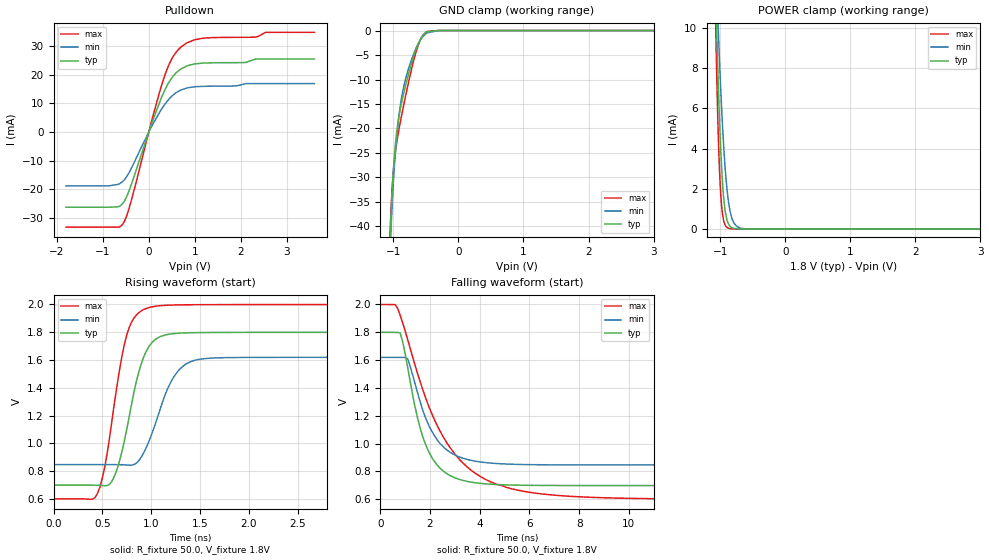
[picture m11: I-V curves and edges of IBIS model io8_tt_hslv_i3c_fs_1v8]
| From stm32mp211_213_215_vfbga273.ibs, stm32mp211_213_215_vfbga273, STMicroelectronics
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[Model]   io8_tt_hslv_i3c_fs_1v8
Model_type I/O_open_drain
Polarity   Non-Inverting
Enable   Active-Low
| CAP_THRESHOLD on pad IOTT is "UDTCAPC" :
| Rising=30.0% of vddiov33m   Falling=70.0% of vddiov33m
| C_comp min and max val. don't necessarily correlate with the min and max pvt
| but are the smallest and greatest pad capacitance found.
| var   typ   min   max
C_comp   1.23130pF  1.11695pF  1.38090pF
|C_comp_pulldown   1.23130pF  1.11695pF  1.38090pF
Vinl = 810.0mV
Vinh = 1.0V
Vmeas = 900.0mV   | Reference voltage for timing measurements
Cref  = 50.0pF   | Timing specification test load capacitance value
Rref  = 1.0MOhm   | Timing specification test load resistance value
Vref  = 990.0mV   | Timing specification test load voltage
[Model Spec]
| TIME_THRESHOLD on pin ZIV08M is "CMOS" :
| Rising=50.0% of vddv08m   Falling=50.0% of vddv08m
Vinl 675.70000mV 623.70000mV 735.70000mV
Vinh 1.12730V 1.01130V 1.24930V
| variable   typ   min   max
[Temperature Range] 25.0 125.0 -40.0
| variable   typ   min   max
[Voltage Range] 1.8V 1.62V 2.0V
| variable   typ   min   max
[POWER Clamp Reference] 1.8V 1.62V 2.0V
| variable   typ   min   max
[GND Clamp Reference] 0V 0V 0V
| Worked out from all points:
|   slope of the pulldown table from 0 to 0.27 V, typ, clamps not added: 22.9 ohm
|   GND clamp passes 1 mA (typ) near -0.55 V on its own axis
|   POWER clamp passes 1 mA (typ) near -0.93 V on its own axis
|   rising waveform, R_fixture 50.0, V_fixture 1.8V: 20-80 % time 209ps typ, 251ps min, 191ps max; typ from 0.698 V to 1.8 V
|   falling waveform, R_fixture 50.0, V_fixture 1.8V: 20-80 % time 948ps typ, 1.06ns min, 2.08ns max; typ from 1.8 V to 0.698 V
[POWER Clamp]
-1.8V     152.1mA    105.6mA    221.1mA
-1.07V    12.07mA    13.61mA    10.38mA
-1.05V    9.569mA    11.75mA    7.248mA
-1.03V    7.339mA    9.993mA    4.743mA
-1.01V    5.42mA     8.357mA    2.898mA
-990mV    3.841mA    6.859mA    1.662mA
-970mV    2.609mA    5.513mA    906.4uA
-940mV    1.358mA    3.806mA    344.1uA
-880mV    308.2uA    1.548mA    45.5uA
-790mV    28.46uA    298.8uA    2.106uA
-610mV    211.8nA    7.522uA    9.52nA
3.6V      0A         0A         0A
[GND Clamp]
-1.8V     -1.222A    -1.193A    -1.238A
-1.05V    -42.33mA   -45.55mA   -41.2mA
-1.04V    -38.89mA   -42.1mA    -37.88mA
-1.03V    -35.83mA   -38.98mA   -35.06mA
-1.01V    -30.7mA    -33.54mA   -30.61mA
-970mV    -23.47mA   -25.17mA   -24.97mA
-920mV    -18.06mA   -18.06mA   -20.63mA
-870mV    -14.51mA   -13.44mA   -17.13mA
-780mV    -9.532mA   -8.354mA   -11.38mA
-650mV    -3.743mA   -3.581mA   -4.327mA
-490mV    -324.1uA   -556uA     -259.6uA
3.6V      66.06nA    2.767uA    18.5nA
| variable   typ   min   max
[Pullup Reference] 1.8V 1.62V 2.0V
| variable   typ   min   max
[Pulldown Reference] 0V 0V 0V
[Pulldown]
-1.8V     -26.25mA   -18.79mA   -33.2mA
-680mV    -26.1mA    -18.31mA   -33.2mA
-550mV    -24.6mA    -16.98mA   -31.75mA
-400mV    -19.26mA   -13.3mA    -25.07mA
70mV      3.286mA    2.202mA    4.389mA
320mV     13.66mA    9.041mA    18.43mA
500mV     18.91mA    12.52mA    25.54mA
700mV     22.05mA    14.7mA     29.73mA
1.18V     24.11mA    15.98mA    32.81mA
2.31V     25.46mA    16.93mA    33.16mA
2.54V     25.56mA    16.93mA    34.85mA
3.6V      25.56mA    16.93mA    34.85mA
[Ramp]
dV/dt_r 661.05492mV/208.84677ps 464.20756mV/250.94674ps 840.41292mV/190.16918ps
dV/dt_f 661.09801mV/946.09206ps 464.25805mV/1.05679ns 840.44915mV/2.07536ns
R_load = 50.0
| Removed startup time: 0s 0s 0s  .
| Removed end time: 6.975ns.
[Rising Waveform]
R_fixture   = 50.0
V_fixture   = 1.8V
V_fixture_min = 1.62V
V_fixture_max = 2.0V
0s        698.2mV    846.2mV    599.3mV
450ps     697.7mV    846.3mV    638.1mV
525ps     694mV      846.3mV    829.9mV
600ps     728.8mV    846.2mV    1.17V
750ps     1.1V       843.4mV    1.78V
875ps     1.517V     876.4mV    1.942V
975ps     1.695V     1.009V     1.977V
1.225ns   1.79V      1.47V      1.996V
1.5ns     1.798V     1.606V     1.998V
6.975ns   1.8V       1.62V      2V
| Removed startup time: 0s 0s 0s  .
| Removed end time: 199.9ns.
[Falling Waveform]
R_fixture   = 50.0
V_fixture   = 1.8V
V_fixture_min = 1.62V
V_fixture_max = 2.0V
0s        1.8V       1.62V      2V
600ps     1.799V     1.62V      1.999V
800ps     1.795V     1.62V      1.922V
1.1ns     1.548V     1.61V      1.748V
1.7ns     1.054V     1.245V     1.391V
2.6ns     793.4mV    965.7mV    1.028V
3.5ns     728mV      885.9mV    831.2mV
4.6ns     706.5mV    857.6mV    713.3mV
8.3ns     698.3mV    846.5mV    615mV
199.9ns   698.2mV    846.2mV    599.3mV
